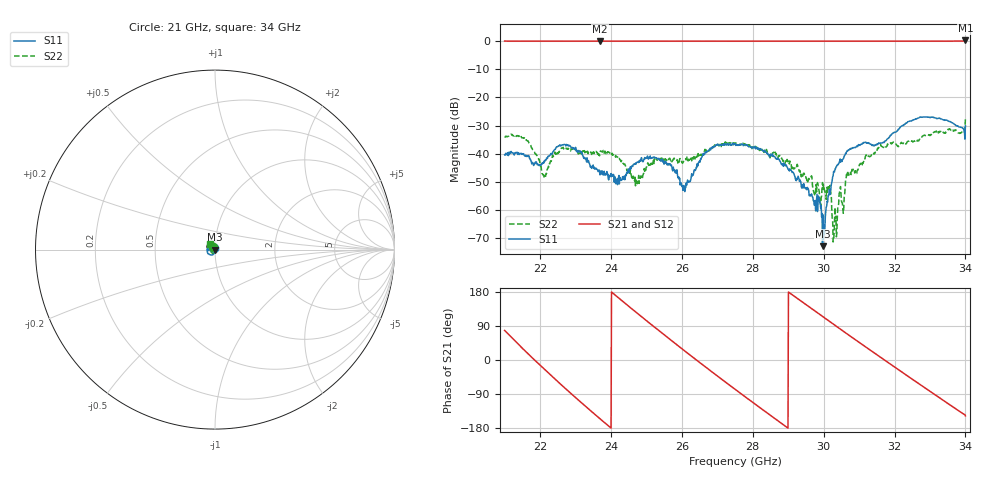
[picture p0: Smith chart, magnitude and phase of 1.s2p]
! 3/6/2025 3:16:31 PM
! C:\USERS\VECTORSTARUSER\DESKTOP\NEW FOLDER\1.S2P
! CHANNEL.1
! TR.MEASUREMENT
! CORRECTED.DATA
! RF.CORRECTION: FULL.TWO.PORT.CAL.PORT.1.2
! AVERAGING.OFF
! IF.BANDWIDTH: NO.IFBW
! SWEEPTYPE:  FREQ.SWEEP(Linear)
! Reference Plane Port Info
! PORT:  PORT1  PORT2
! DISTANCE:  0  m  0  m
! TIME:  0  s  0  s
! PHASE.OFFSET:  0 °  0 °
! LOSS:  0  dB  0  dB
! REF.LOSS:  0  dB  0  dB
! REF.FREQ:  0  Hz  0  Hz
! Power Info
! POWER:  -10  dBm  -10  dBm
! EFF.POWER:  -10  dBm  -10  dBm
! SOURCE.ATTEN:  0  dB  0  dB
! TEST.ATTEN:  0  dB  0  dB
# GHZ S RI R 50.0
! FREQ.GHZ  S11RE  S11IM  S21RE  S21IM  S12RE  S12IM  S22RE  S22IM
!; PortSelection: Port_12
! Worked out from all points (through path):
!   1001 points, 21 GHz to 34 GHz, reference 50 ohm
!   highest |S21| = 0.19 dB at 34 GHz (marker M1); lowest = -0.1 dB at 23.69 GHz (marker M2)
!   lowest |S11| = -72.7 dB at 29.97 GHz (marker M3), VSWR 1.00, Z = 50 - j0.0208 ohm
!   |S11| at or under -10 dB: start of sweep to end of sweep
!   |S22| runs from -71.3 to -27.8 dB; largest |S21 - S12| = 0.0039
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21  -0.00659 0.00702  0.2053 0.9763  0.2046 0.9749  -0.0118 0.0161
21.533  -0.0048 0.00883  0.8788 0.4678  0.8753 0.4694  0.00471 0.0182
21.975  -0.00411 0.00458  0.9751 -0.1985  0.9747 -0.1988  0.00584 0.00534
22.118  -0.00686 0.00293  0.9087 -0.4074  0.9067 -0.4071  0.00158 0.00339
22.612  -0.0109 0.00932  0.3953 -0.9131  0.3961 -0.9127  0.0034 0.0122
23.171  -0.00345 0.0103  -0.3881 -0.9152  -0.3901 -0.9148  0.00429 0.00927
23.691  -0.00202 0.00371  -0.8984 -0.4209  -0.9012 -0.4224  0.00833 0.00617
24.198  -0.0032 0.00129  -0.9612 0.2548  -0.9625 0.2551  0.00858 -0.00062
24.705  -0.00656 -0.000544  -0.5874 0.8031  -0.5857 0.8037  -0.000972 -0.00331
25.342  -0.00789 0.00257  0.2032 0.9749  0.2025 0.9752  -0.00525 0.00634
26.044  -0.00258 0.00062  0.8887 0.4469  0.8897 0.4456  0.00637 0.00359
26.408  -0.00378 -0.00442  0.9951 0.00454  0.9941 0.00492  0.00773 -0.00388
27.5  -0.0152 0.00142  0.2231 -0.9698  0.2221 -0.9685  -0.0111 -0.0108
28.683  -0.00545 0.00626  -0.9253 -0.3618  -0.9263 -0.3636  -0.000668 0.00937
29.671  -0.00158 0.000953  -0.7006 0.7082  -0.7009 0.7063  0.00359 -0.00134
29.97  -9.81e-05 -0.000208  -0.4178 0.9055  -0.4172 0.9053  -0.0016 -0.00265
30.152  0.00172 -0.00101  -0.2176 0.9728  -0.2173 0.9734  -0.000913 -0.00199
30.321  0.00341 -0.00412  -0.0248 0.9973  -0.0249 0.9962  -0.00109 -0.000276
30.698  0.00127 -0.0115  0.3969 0.9149  0.3957 0.9145  0.00249 0.00341
31.842  -0.00456 -0.0187  0.986 -0.1405  0.986 -0.141  0.00192 -0.0148
32.96  -0.0437 -0.01  0.1727 -0.9792  0.1732 -0.9798  -0.0127 -0.0174
34  -0.0287 0.0127  -0.8613 -0.5509  -0.8603 -0.5501  -0.0278 0.03
